(* Logix 5000 Rung export; software revision 29.00 *)

VAR_GLOBAL   (* controller tags *)
   CopyNMCmdToSend : BOOL;
   msg_NMCmd : MESSAGE;
        MessageParameters(MessageType := CIP Generic, RequestedLength := 14, ConnectedFlag := 2, ConnectionPath := is5705, ServiceCode := 16#0034, ObjectType := 16#0078, TargetObject := 1, LocalElement := SendNM_Cmd.DATA[0], DestinationTag := NMCmd_ResultString.DATA[0])
   NativeModeCmds : STRING[20] := ([0] := 'SO0', [1] := 'GO', [2] := 'TFEIP_NM_Auto-Stored.job', [3] := 'GF', [4] := 'LFEIP_NM_Auto.job', [5] := 'SO1', [6] := 'GO');
   NMCmd_ResultString : STRING;
   NMCmdIndx : COUNTER := (PRE := 7);
   SendNM_Cmd : STRING := 'SO0';
END_VAR

PROGRAM MainProgram
VAR
   send_NMCmd : BOOL;
END_VAR

ROUTINE MainRoutine   (* ladder *)
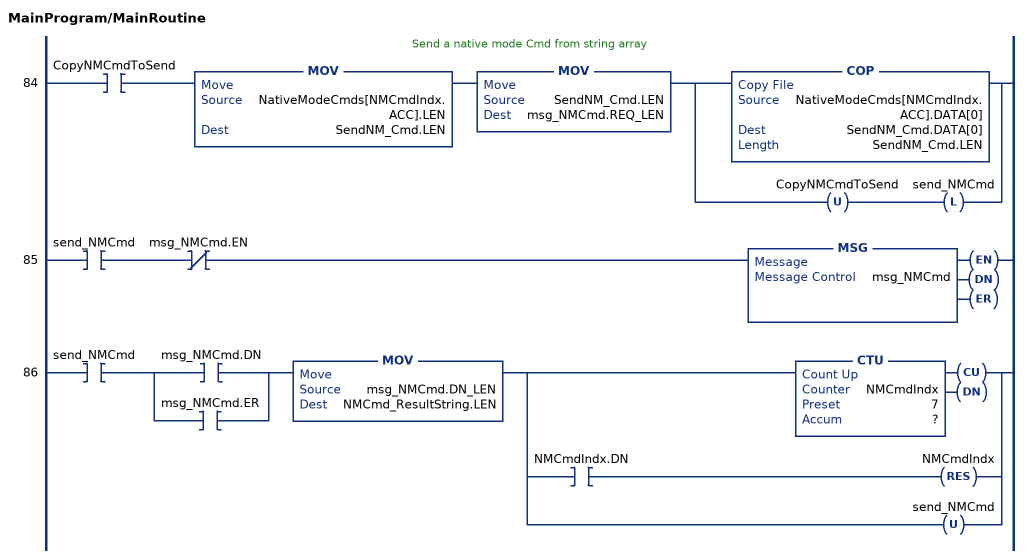
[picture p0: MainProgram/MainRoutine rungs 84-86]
   // Send a native mode Cmd from string array
   84: XIC(CopyNMCmdToSend)MOV(NativeModeCmds[NMCmdIndx.ACC].LEN,SendNM_Cmd.LEN)MOV(SendNM_Cmd.LEN,msg_NMCmd.REQ_LEN)[COP(NativeModeCmds[NMCmdIndx.ACC].DATA[0],SendNM_Cmd.DATA[0],SendNM_Cmd.LEN) ,OTU(CopyNMCmdToSend) OTL(send_NMCmd) ];
   85: XIC(send_NMCmd)XIO(msg_NMCmd.EN)MSG(msg_NMCmd);
   86: XIC(send_NMCmd)[XIC(msg_NMCmd.DN) ,XIC(msg_NMCmd.ER) ]MOV(msg_NMCmd.DN_LEN,NMCmd_ResultString.LEN)[CTU(NMCmdIndx,?,?) ,XIC(NMCmdIndx.DN) RES(NMCmdIndx) ,OTU(send_NMCmd) ];
END_ROUTINE
END_PROGRAM
